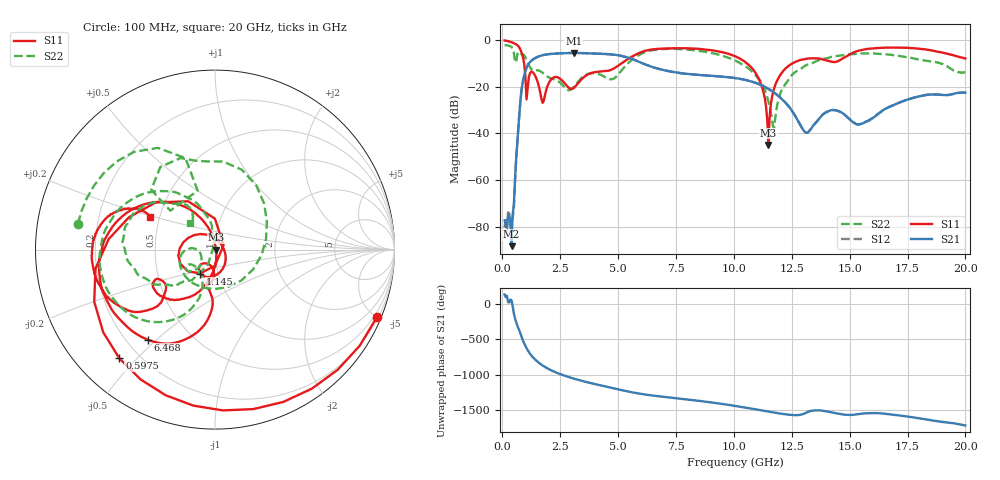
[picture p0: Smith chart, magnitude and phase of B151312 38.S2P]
!  2-Port S-parameters saved by WinCal
! VAR MeasName=S-Parameters (CALIBRATED_DATA) read from VNA (N5244A)
! VAR MeasDate=12/8/2015 5:46:37 PM
! VAR NAME=B151312 38
! VAR FILENAME=B151312 38.S2P
! VAR DATE=12/8/2015 5:46:37 PM
! VAR PHYS_PORTS=1,2
# Hz S DB R 50
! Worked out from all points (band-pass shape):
!   401 points, 100 MHz to 20 GHz, reference 50 ohm
!   highest |S21| = -5.54 dB at 3.085 GHz (marker M1); lowest = -88.4 dB at 398.5 MHz (marker M2)
!   |S21| within 3 dB of the highest: 1.298 GHz to 5.703 GHz (4.405 GHz wide, 126 % of centre)
!   lowest |S11| = -45.1 dB at 11.49 GHz (marker M3), VSWR 1.01, Z = 50.5 - j0.119 ohm
!   |S11| at or under -10 dB: 941.6 MHz to 5.159 GHz (4.217 GHz wide, 138 % of centre); 10.56 GHz to 12.53 GHz (1.971 GHz wide, 17.1 % of centre)
!   |S22| runs from -37.6 to -2.2 dB; largest |S21 - S12| = 0.0016
!   S11 on the Smith chart (normalised r, x): 100 MHz: 0.29, -4.99; 597.5 MHz: 0.13, -0.45; 1.145 GHz: 0.82, -0.22; 6.468 GHz: 0.28, -0.47; 20 GHz: 0.45, +0.19
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1e8  -0.20 -22.6  -77.37 134.5  -80.52 -129.0  -2.19 169.3
3.985e8  -0.94 -87.2  -88.43 54.6  -79.07 -19.2  -3.02 129.6
5.975e8  -1.86 -131.3  -51.33 105.7  -51.05 105.2  -9.63 139.0
8.4625e8  -5.82 159.4  -20.28 -119.1  -20.28 -119.1  -6.13 95.4
1.14475e9  -16.08 -122.0  -10.08 41.1  -10.08 41.1  -10.72 12.1
1.493e9  -17.01 145.0  -7.40 -88.6  -7.39 -88.6  -12.98 -123.5
1.74175e9  -26.95 38.8  -6.53 -150.1  -6.53 -150.1  -14.08 -167.8
1.94075e9  -20.03 -56.9  -6.14 170.4  -6.14 170.4  -15.67 -178.3
2.43825e9  -16.22 -122.8  -5.75 95.5  -5.75 95.5  -17.78 176.7
3.085e9  -20.60 -104.0  -5.54 24.4  -5.55 24.4  -20.12 -139.0
3.43325e9  -16.71 -92.1  -5.61 -7.6  -5.61 -7.6  -16.17 -133.9
4.52775e9  -13.28 -101.2  -6.05 -92.9  -6.04 -92.8  -16.43 -145.8
6.468e9  -4.06 -126.7  -11.57 145.5  -11.52 145.3  -4.40 -144.5
6.7665e9  -3.78 -135.2  -12.41 133.7  -12.41 133.6  -3.98 -155.1
1.005e10  -6.95 144.7  -16.33 -2.2  -16.33 -2.3  -8.75 122.2
1.1045e10  -16.00 110.6  -18.77 -57.5  -18.78 -57.5  -16.25 99.1
1.149275e10  -45.06 -12.1  -20.96 -83.3  -20.94 -83.2  -26.26 95.7
1.17415e10  -20.69 -89.3  -22.55 -97.4  -22.55 -97.3  -37.59 -175.8
1.204e10  -14.47 -103.0  -25.05 -113.0  -25.01 -113.1  -22.07 -116.5
1.338325e10  -7.85 -144.8  -37.40 -70.1  -37.40 -70.4  -9.89 -141.5
1.67165e10  -3.28 -171.7  -28.73 -121.2  -28.62 -122.0  -6.27 153.6
2e10  -7.92 153.5  -22.59 80.5  -22.65 80.2  -13.94 133.0
